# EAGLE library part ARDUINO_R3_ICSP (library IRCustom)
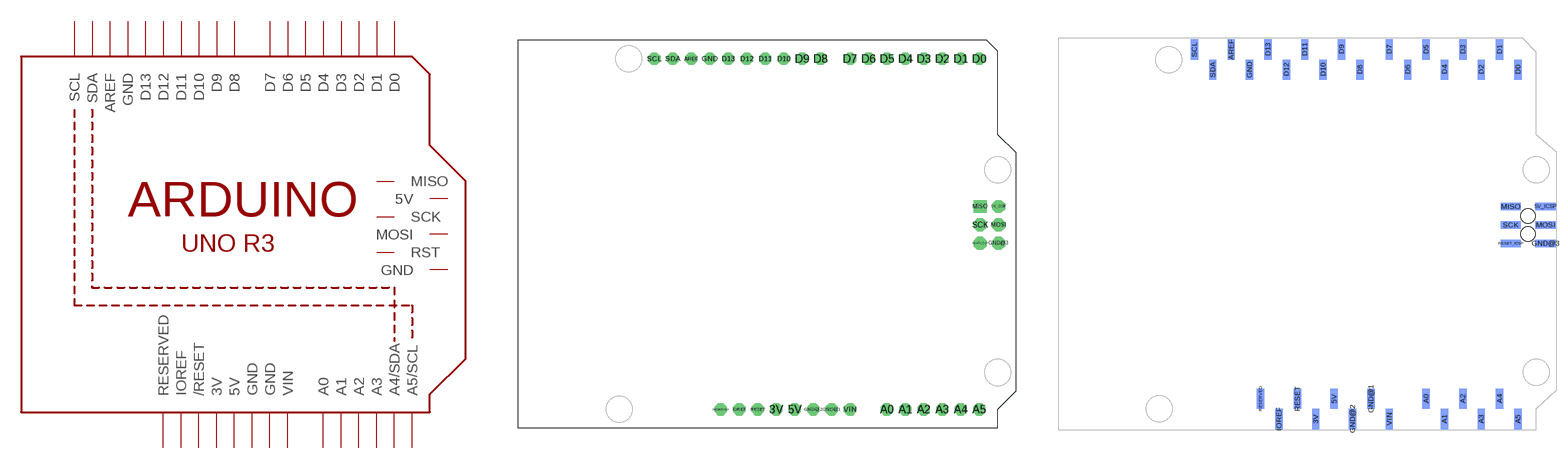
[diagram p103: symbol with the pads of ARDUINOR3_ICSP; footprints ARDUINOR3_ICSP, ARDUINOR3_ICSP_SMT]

Designator prefix M

## ARDUINO_R3_ICSP  [ARDUINOR3_ICSP]
3V  3V  pwr
5V  5V  pwr
5V_ICSP  5V  pas
A0  A0
A1  A1
A2  A2
A3  A3
A4  A4/SDA
A5  A5/SCL
AREF  AREF
D0  D0
D1  D1
D2  D2
D3  D3
D4  D4
D5  D5
D6  D6
D7  D7
D8  D8
D9  D9
D10  D10
D11  D11
D12  D12
D13  D13
GND  GND  pwr
GND@1  GND  pwr
GND@2  GND  pas
GND@3  GND  pwr
IOREF  IOREF  out
MISO  MISO  pas
MOSI  MOSI  pas
RESERVED  RESERVED  nc
RESET  /RESET
RESET_ICSP  RST  pas
SCK  SCK  pas
SCL  SCL
SDA  SDA
VIN  VIN  pwr

## ARDUINO_R3_ICSPSMT  [ARDUINOR3_ICSP_SMT]
3V  3V  pwr
5V  5V  pwr
5V_ICSP  5V  pas
A0  A0
A1  A1
A2  A2
A3  A3
A4  A4/SDA
A5  A5/SCL
AREF  AREF
D0  D0
D1  D1
D2  D2
D3  D3
D4  D4
D5  D5
D6  D6
D7  D7
D8  D8
D9  D9
D10  D10
D11  D11
D12  D12
D13  D13
GND  GND  pwr
GND@1  GND  pwr
GND@2  GND  pwr
GND@3  GND  pas
IOREF  IOREF  out
MISO  MISO  pas
MOSI  MOSI  pas
RESERVED  RESERVED  nc
RESET  /RESET
RESET_ICSP  RST  pas
SCK  SCK  pas
SCL  SCL
SDA  SDA
VIN  VIN  pwr

## ARDUINO_R3_ICSP_NODIM  [ARDUINOR3_ICSP_NODIM]
Pads as for ARDUINOR3_ICSP

## Footprint ARDUINOR3_ICSP (pad centres in mm)
drill 1 pad 1.676 octagon: 3V 35.56,2.54; 5V 38.1,2.54; A0 50.8,2.54; A1 53.34,2.54; A2 55.88,2.54; A3 58.42,2.54; A4 60.96,2.54; A5 63.5,2.54; AREF 23.876,50.8; D0 63.5,50.8; D1 60.96,50.8; D2 58.42,50.8; D3 55.88,50.8; D4 53.34,50.8; D5 50.8,50.8; D6 48.26,50.8; D7 45.72,50.8; D8 41.656,50.8; D9 39.116,50.8; D10 36.576,50.8; D11 34.036,50.8; D12 31.496,50.8; D13 28.956,50.8; GND 26.416,50.8; GND@1 43.18,2.54; GND@2 40.64,2.54; IOREF 30.48,2.54; RESERVED 27.94,2.54; RESET 33.02,2.54; SCL 18.796,50.8; SDA 21.336,50.8; VIN 45.72,2.54
drill 1 pad 1.778 octagon: 5V_ICSP 66.167,30.48; GND@3 66.167,25.4; MOSI 66.167,27.94; RESET_ICSP 63.627,25.4; SCK 63.627,27.94
drill 1 pad 1.778 square: MISO 63.627,30.48

## Footprint ARDUINOR3_ICSP_SMT (pad centres in mm)
smd 1.016 x 2.794 bottom: 3V 35.56,1.143; 5V 38.1,3.937; A0 50.8,3.937; A1 53.34,1.143; A2 55.88,3.937; A3 58.42,1.143; A4 60.96,3.937; A5 63.5,1.143; AREF 23.876,52.197; D0 63.5,49.403; D1 60.96,52.197; D2 58.42,49.403; D3 55.88,52.197; D4 53.34,49.403; D5 50.8,52.197; D6 48.26,49.403; D7 45.72,52.197; D8 41.656,49.403; D9 39.116,52.197; D10 36.576,49.403; D11 34.036,52.197; D12 31.496,49.403; D13 28.956,52.197; GND 26.416,49.403; GND@1 43.18,3.937; GND@2 40.64,1.143; IOREF 30.48,1.143; RESERVED 27.94,3.937; RESET 33.02,3.937; SCL 18.796,52.197; SDA 21.336,49.403; VIN 45.72,1.143
smd 2.794 x 1.016 bottom: 5V_ICSP 67.31,30.48; GND@3 67.31,25.4; MISO 62.484,30.48; MOSI 67.31,27.94; RESET_ICSP 62.484,25.4; SCK 62.484,27.94
hole 2 at 64.897,29.21
hole 2 at 64.897,26.67

## Footprint ARDUINOR3_ICSP_NODIM (pad centres in mm)
drill 1 pad 1.676 octagon: 3V 35.56,2.54; 5V 38.1,2.54; A0 50.8,2.54; A1 53.34,2.54; A2 55.88,2.54; A3 58.42,2.54; A4 60.96,2.54; A5 63.5,2.54; AREF 23.876,50.8; D0 63.5,50.8; D1 60.96,50.8; D2 58.42,50.8; D3 55.88,50.8; D4 53.34,50.8; D5 50.8,50.8; D6 48.26,50.8; D7 45.72,50.8; D8 41.656,50.8; D9 39.116,50.8; D10 36.576,50.8; D11 34.036,50.8; D12 31.496,50.8; D13 28.956,50.8; GND 26.416,50.8; GND@1 43.18,2.54; GND@2 40.64,2.54; IOREF 30.48,2.54; RESERVED 27.94,2.54; RESET 33.02,2.54; SCL 18.796,50.8; SDA 21.336,50.8; VIN 45.72,2.54
drill 1 pad 1.778 octagon: 5V_ICSP 66.167,30.48; GND@3 66.167,25.4; MOSI 66.167,27.94; RESET_ICSP 63.627,25.4; SCK 63.627,27.94
drill 1 pad 1.778 square: MISO 63.627,30.48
